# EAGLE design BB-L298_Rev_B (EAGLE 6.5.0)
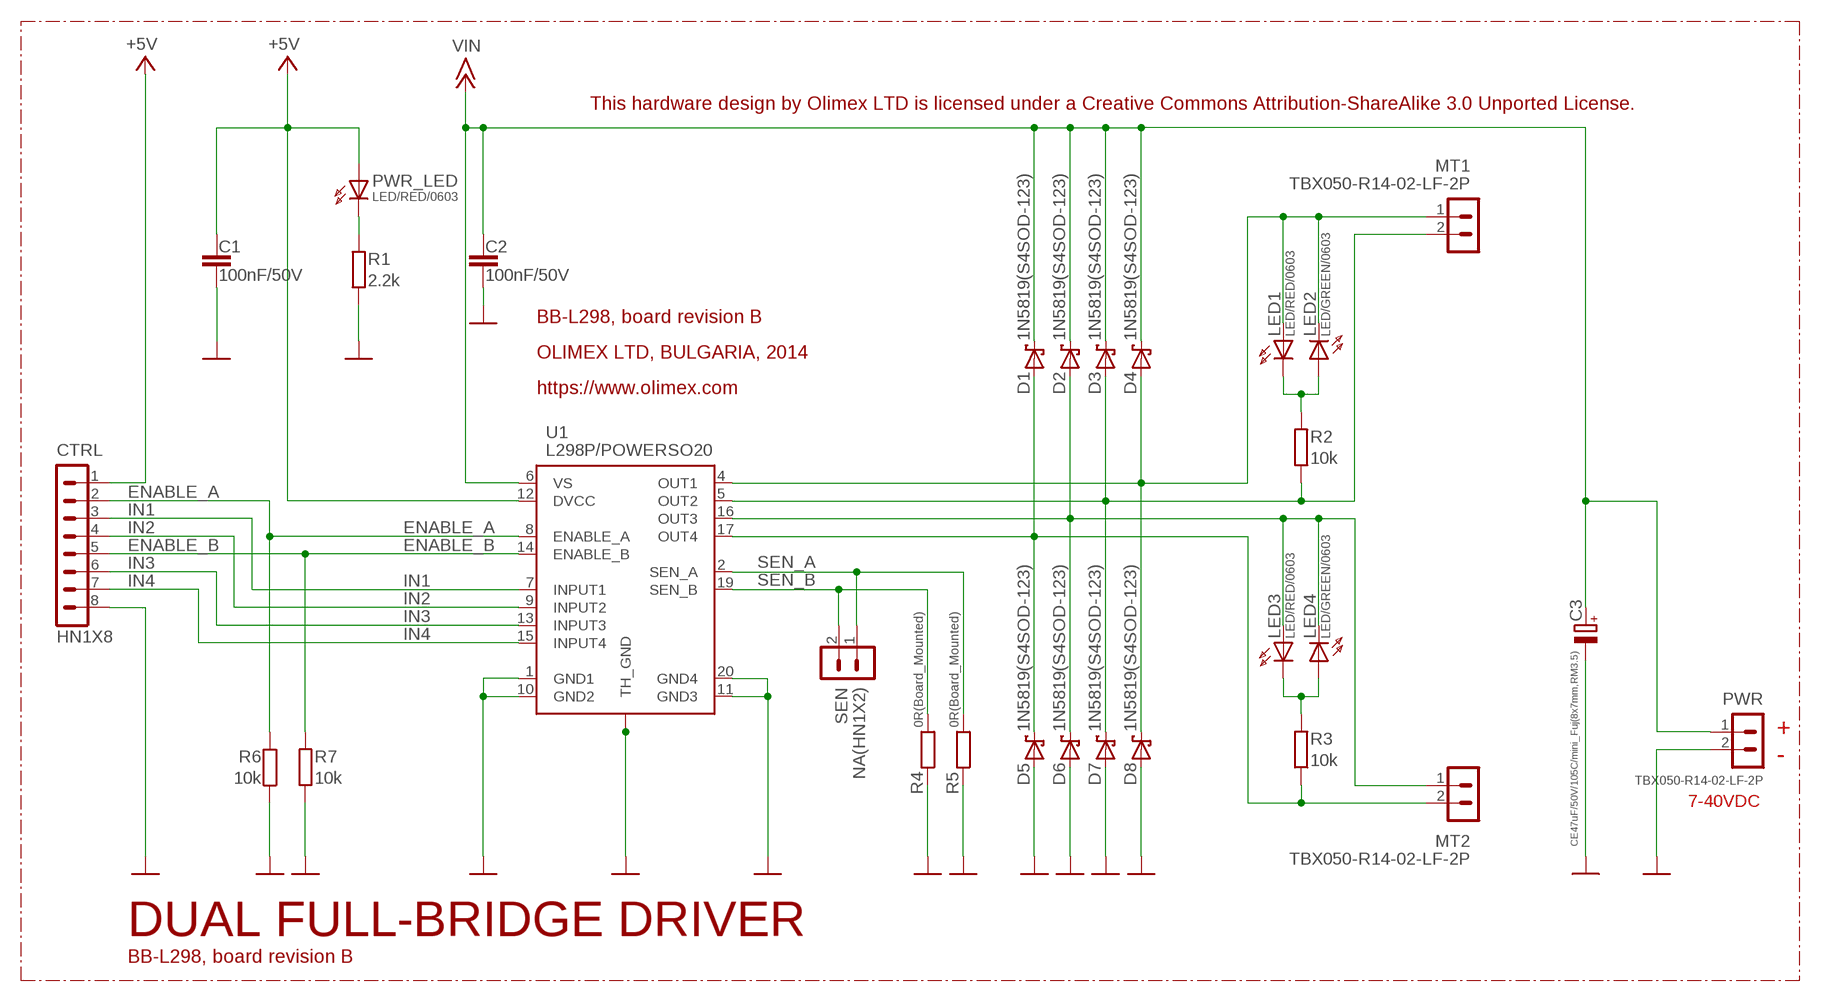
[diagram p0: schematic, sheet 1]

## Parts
C1  100nF/50V  C-EUC0603_DWS  [C0603_DWS]
C2  100nF/50V  C-EUC0603_DWS  [C0603_DWS]
C3  CE47uF/50V/105C/mini_Fuj(8x7mm,RM3.5)  CPOL-EUE3.5-8  [E3,5-8]
CTRL  HN1X8  CON8HN1X8  [HN1X8]
D1  1N5819(S4SOD-123)  SCHOTKKY7.62SS-1N5819(S4SOD-123)  [SOD-123]
D2  1N5819(S4SOD-123)  SCHOTKKY7.62SS-1N5819(S4SOD-123)  [SOD-123]
D3  1N5819(S4SOD-123)  SCHOTKKY7.62SS-1N5819(S4SOD-123)  [SOD-123]
D4  1N5819(S4SOD-123)  SCHOTKKY7.62SS-1N5819(S4SOD-123)  [SOD-123]
D5  1N5819(S4SOD-123)  SCHOTKKY7.62SS-1N5819(S4SOD-123)  [SOD-123]
D6  1N5819(S4SOD-123)  SCHOTKKY7.62SS-1N5819(S4SOD-123)  [SOD-123]
D7  1N5819(S4SOD-123)  SCHOTKKY7.62SS-1N5819(S4SOD-123)  [SOD-123]
D8  1N5819(S4SOD-123)  SCHOTKKY7.62SS-1N5819(S4SOD-123)  [SOD-123]
LED1  LED/RED/0603  LED0603DWS  [LED-0603]
LED2  LED/GREEN/0603  LED0603DWS  [LED-0603]
LED3  LED/RED/0603  LED0603DWS  [LED-0603]
LED4  LED/GREEN/0603  LED0603DWS  [LED-0603]
MT1  TBX050-R14-02-LF-2P  CON2_TBX050-R14-02-LF-2P  [TBX050-R14-02-LF-2P]
MT2  TBX050-R14-02-LF-2P  CON2_TBX050-R14-02-LF-2P  [TBX050-R14-02-LF-2P]
PWR  TBX050-R14-02-LF-2P  CON2_TBX050-R14-02-LF-2P  [TBX050-R14-02-LF-2P]
PWR_LED  LED/RED/0603  LED0603DWS  [LED-0603]
R1  2.2k  R-EU_R0603_5MIL_DWS  [R0603_5MIL_DWS]
R2  10k  R-EU_R0603_5MIL_DWS  [R0603_5MIL_DWS]
R3  10k  R-EU_R0603_5MIL_DWS  [R0603_5MIL_DWS]
R4  0R(Board_Mounted)  R-EU_R1206_5MIL_WS  [R1206_5MIL_WS]
R5  0R(Board_Mounted)  R-EU_R1206_5MIL_WS  [R1206_5MIL_WS]
R6  10k  R-EU_R0603_5MIL_DWS  [R0603_5MIL_DWS]
R7  10k  R-EU_R0603_5MIL_DWS  [R0603_5MIL_DWS]
SEN  NA(HN1X2)  CON2HN1X2  [HN1X2]
U1  L298P/POWERSO20  [POWRESO-20_THERM]

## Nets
+5V: C1.2 CTRL.1 PWR_LED.A U1.12(DVCC)
+15V: C2.2 C3.+ D1.C D2.C D3.C D4.C PWR.1 U1.6(VS) ; supply symbol labelled VIN
ENABLE_A: CTRL.2 R6.2 U1.8(ENABLE_A)
ENABLE_B: CTRL.5 R7.2 U1.14(ENABLE_B)
GND [pwr]: C1.1 C2.1 C3.- CTRL.8 D5.A D6.A D7.A D8.A PWR.2 R1.1 R4.1 R5.1 R6.1 R7.1 U1.1(GND1) U1.10(GND2) U1.11(GND3) U1.20(GND4) U1.THERM_GND1(TH_GND) U1.THERM_GND2 U1.THERM_GND3 U1.THERM_GND4 U1.THERM_GND5 U1.THERM_GND6 U1.THERM_GND7
IN1: CTRL.3 U1.7(INPUT1)
IN2: CTRL.4 U1.9(INPUT2)
IN3: CTRL.6 U1.13(INPUT3)
IN4: CTRL.7 U1.15(INPUT4)
N$1: LED1.C LED2.A R2.2
N$2: LED3.C LED4.A R3.2
N$3: PWR_LED.C R1.2
OUT1: D4.A D8.C LED1.A LED2.C MT1.1 U1.4(OUT1)
OUT2: D3.A D7.C MT1.2 R2.1 U1.5(OUT2)
OUT3: D2.A D6.C LED3.A LED4.C MT2.1 U1.16(OUT3)
OUT4: D1.A D5.C MT2.2 R3.1 U1.17(OUT4)
SEN_A: R5.2 SEN.1 U1.2(SEN_A)
SEN_B: R4.2 SEN.2 U1.19(SEN_B)

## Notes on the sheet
- This hardware design by Olimex LTD is licensed under a Creative Commons Attribution-ShareAlike 3.0 Unported License.
- BB-L298, board revision B
- OLIMEX LTD, BULGARIA, 2014
- https://www.olimex.com
- +
- -
- 7-40VDC
- DUAL FULL-BRIDGE DRIVER
- BB-L298, board revision B

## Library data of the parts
C1 C2 = rcl:C-EU: CAPACITOR, European symbol
C3 = rcl:CPOL-EU: POLARIZED CAPACITOR, European symbol
CTRL = Penko:CON8
D1-D8 = gogo:SCHOTKKY7.62SS
LED1-LED4 PWR_LED = DOUBLE-SIDE:LED
MT1 MT2 PWR SEN = Penko:CON2
R1-R7 = rcl:R-EU_: RESISTOR, European symbol
U1 = st-microelectronics:L298P

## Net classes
0 default: width 0.254 mm, drill 0.6 mm, clearance 0.254 mm
1 pwr: width 0.25 mm
2 thin: width 0.025 mm, clearance 0.025 mm
3 gsm_pwr: width 0.914 mm, drill 0.787 mm

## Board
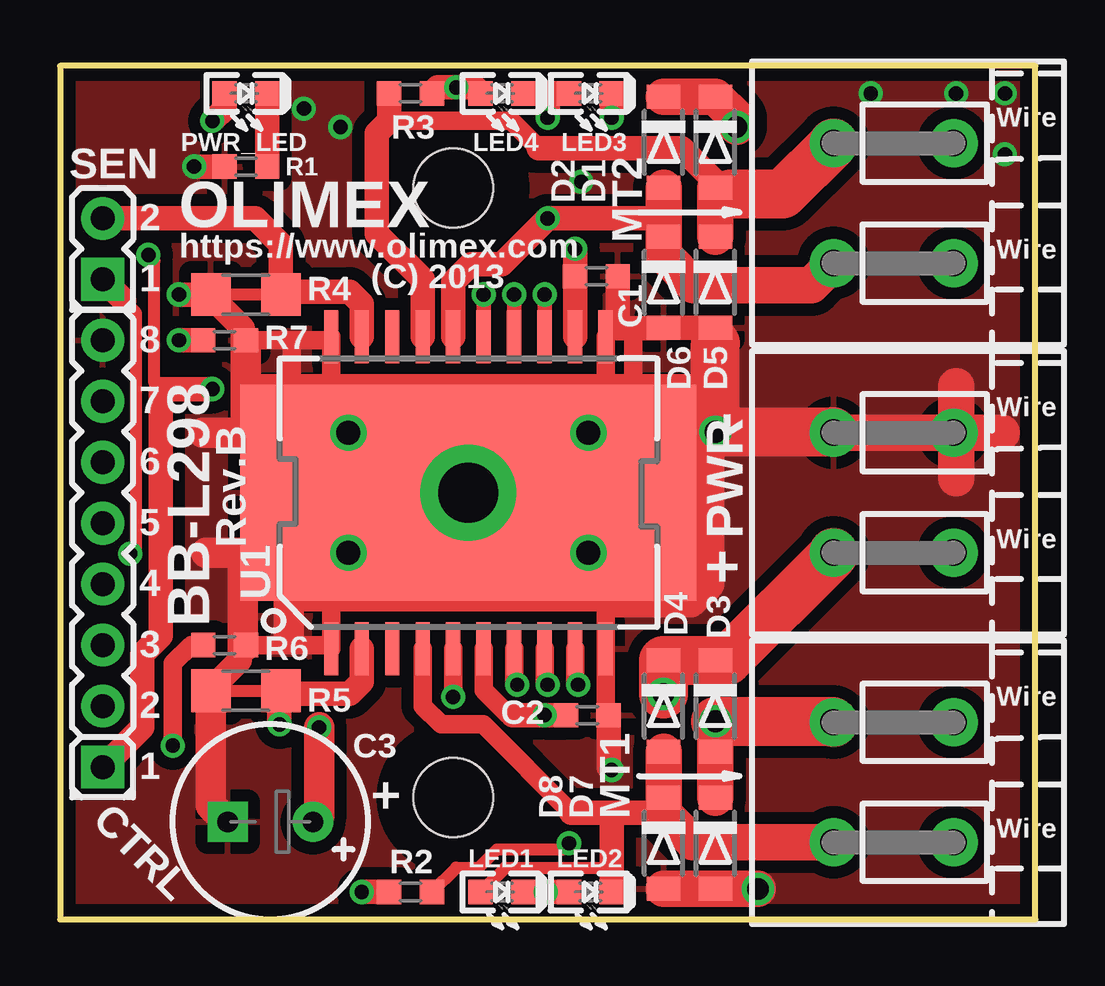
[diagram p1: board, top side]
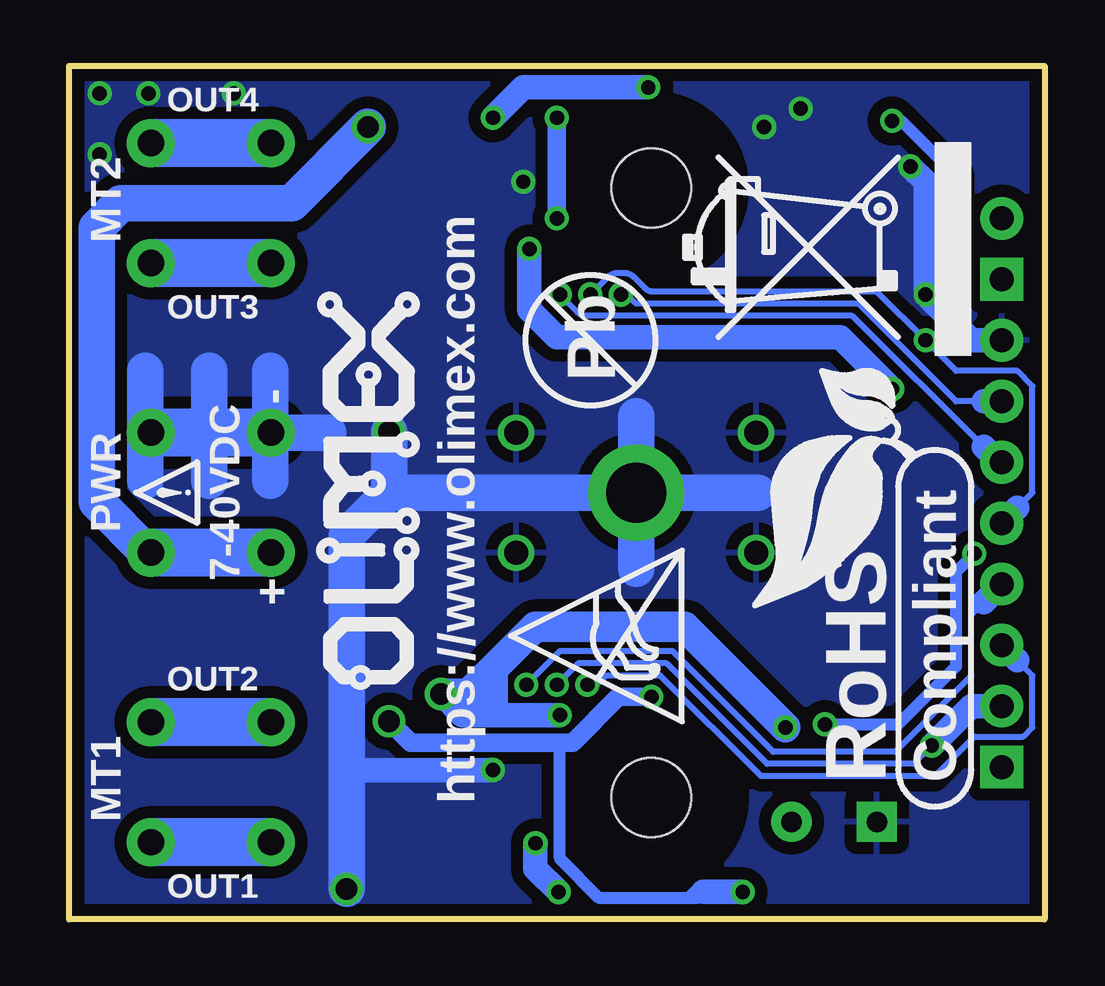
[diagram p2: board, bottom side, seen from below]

Size 40.64 x 35.56 mm. Coordinates in mm from the lower left corner, seen from the top.
Outline: 0,0 40.64,0 40.64,35.56 0,35.56 0,0
Copper layers (1+16): Top 0.035mm / dielectric 1.5mm / Bottom 0.035mm
Design rules "default": minimum track width 9.5mil, minimum drill 23mil, track to track 9.5mil, track to pad 9.5mil, pad to pad 9.5mil, via to via 10mil, smd to smd 1mil, copper to edge 10mil, drill to drill 8mil, minimum pad ring 10mil, minimum via ring 8mil, stop-mask expansion 4mil, vias tented up to drill 40mil, thermal gap 20mil
Holes 3.3 mm at 16.38,30.48 16.38,5.08
tRestrict: area 13.8,27.9 to 18.9,33; area 13.8,2.5 to 18.9,7.6; 2 lines
bRestrict: area 13,27.1 to 19.8,33.9; area 13,1.7 to 19.8,8.5

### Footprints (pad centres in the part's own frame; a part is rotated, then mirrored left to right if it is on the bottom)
C0603_DWS = smd 1.016 x 1.016: 1 -0.889,0; 2 0.889,0
E3,5-8 = drill 0.864 pad 1.676: + -1.778,0 | drill 0.864 pad 1.676 square: - 1.778,0
HN1X8 = drill 1 pad 1.778 square: 1 -8.89,0 | drill 1 pad 1.778: 2 -6.35,0; 3 -3.81,0; 4 -1.27,0; 5 1.27,0; 6 3.81,0; 7 6.35,0; 8 8.89,0
SOD-123 = smd 1 x 1.4: A 1.9,0; C -1.9,0
LED-0603 = smd 1.016 x 1.016: A 0.889,0; C -0.889,0
TBX050-R14-02-LF-2P = drill 1.1 pad 2: 1 -2.5,3.2; 2 2.5,3.2; 3 -2.5,-1.8; 4 2.5,-1.8
R0603_5MIL_DWS = smd 1.016 x 1.016: 1 -0.889,0; 2 0.889,0
R1206_5MIL_WS = smd 1.651 x 1.778: 1 -1.46,0; 2 1.46,0
HN1X2 = drill 1 pad 1.778 square: 1 -1.27,0 | drill 1 pad 1.778: 2 1.27,0
POWRESO-20_THERM = smd 0.6 x 2.2: 1 -5.715,-6.5; 2 -4.445,-6.5; 3 -3.175,-6.5; 4 -1.905,-6.5; 5 -0.635,-6.5; 6 0.635,-6.5; 7 1.905,-6.5; 8 3.175,-6.5; 9 4.445,-6.5; 10 5.715,-6.5; 11 5.715,6.5; 12 4.445,6.5; 13 3.175,6.5; 14 1.905,6.5; 15 0.635,6.5; 16 -0.635,6.5; 17 -1.905,6.5; 18 -3.175,6.5; 19 -4.445,6.5; 20 -5.715,6.5 | smd 10 x 9: THERM_GND1 -4.5,0; THERM_GND2 4.5,0 | drill 2.5 pad 4: THERM_GND3 0,0 | drill 1: THERM_GND4 -5,2.5; THERM_GND5 -5,-2.5; THERM_GND6 5,2.5; THERM_GND7 5,-2.5

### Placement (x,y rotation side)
C1  22.35,26.8 180 top
C2  21.97,8.51 180 top
C3  8.76,4.06 180 top
CTRL  1.78,15.24 90 top
D1  27.3,32.38 270 top
D2  25.15,32.38 270 top
D3  27.3,8.89 270 top
D4  25.15,8.89 270 top
D5  27.3,26.54 270 top
D6  25.15,26.54 270 top
D7  27.3,3.17 270 top
D8  25.15,3.17 270 top
LED1  18.42,1.14 180 top
LED2  22.1,1.14 180 top
LED3  22.1,34.42 180 top
LED4  18.42,34.42 180 top
MT1  35.43,5.71 90 top
MT2  35.43,29.84 90 top
PWR  35.43,17.78 90 top
PWR_LED  7.75,34.42 180 top
R1  7.75,31.37 0 top
R2  14.6,1.14 0 top
R3  14.6,34.42 0 top
R4  7.75,26.04 0 top
R5  7.75,9.53 0 top
R6  6.86,11.43 180 top
R7  6.86,24.13 180 top
SEN  1.78,27.94 90 top
U1  17.02,17.78 0 top
U$1  [ATTENTION_SMALL]  35.31,16.51 90 bottom
U$3  [RECYCLE_BIN1/4]  3.05,23.5 90 bottom
U$5  [ESD_SYMBOL]  15.11,8.26 90 bottom
U$6  [PB]  18.92,24.13 90 bottom
U$13  [ROHS]  3.68,5.71 90 bottom
U$14  [OLIMEX1_V]  25.91,27.3 90 bottom

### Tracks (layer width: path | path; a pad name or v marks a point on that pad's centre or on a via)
+5V  (via drill 0.6)
  Top 0.508: 4.19,22.1 3.94,22.35 3.94,27.43 v3.68,27.69
  Top 1.016: U1.12 C1.2 v21.46,27.94 | CTRL.1 3.43,8 3.43,11.05 4.19,11.81 4.19,22.1 v6.35,22.1 | v6.35,33.27 6.86,33.78 PWR_LED.A
  Bottom 0.508: v6.35,33.27 5.97,33.27 3.68,30.99 v3.68,27.69
  Bottom 1.016: v21.46,27.94 21.46,25.4 20.32,24.26 8.51,24.26 v6.35,22.1
+15V  (via drill 0.6, 0.9)
  Top 0.762: U1.6 17.65,9.55 18.69,8.51 18.87,8.51
  Top 1.016: 18.87,8.51 v20.19,8.51 C2.2
  Top 1.27: C3.+ 10.79,4.32 v10.79,8
  Top 1.524: v28.19,33.02 28.19,33.4 D1.C D2.C
  Top 2.032: v25.15,9.4 D4.C D3.C 27.81,10.79 32.23,15.21 PWR.1
  Bottom 0.762: 22.73,10.67 22.73,8.51 23.75,9.53 23.88,9.53
  Bottom 1.016: 23.11,8.51 24,9.4 | 23.11,8.51 22.73,8.51 v20.19,8.51 | 23.11,8.51 24.26,8.51 v25.15,9.4
  Bottom 1.27: v25.15,9.4 24,9.4 23.88,9.53 22.73,10.67 21.21,12.19 14.99,12.19 v10.79,8
  Bottom 1.524: PWR.1 37.38,15.28 39.5,17.4 39.5,28.83 38.48,29.84 31.37,29.84 v28.19,33.02
ENABLE_A  (via drill 0.6)
  Top 0.762: v20.32,9.78 20.19,9.91 U1.8 | R6.2 5.46,11.43 4.7,10.67 v4.7,7.24
  Bottom 0.254: v20.32,9.78 19.43,10.67 15.75,10.67 11.56,6.48 5.46,6.48 v4.7,7.24
  Bottom 1.016: CTRL.2 3.05,8.89 v4.7,7.24
ENABLE_B  (via drill 0.6)
  Top 0.61: v18.92,26.04 U1.14
  Top 1.016: v4.95,24.13 R7.2
  Bottom 0.254: v18.92,26.04 18.18,26.77 arc45 17.82,26.92 17.48,26.92 arc45 17.12,26.77 16.66,26.31 arc-45 16.3,26.16 6.99,26.16 v4.95,24.13 3.68,22.86 1.14,22.86 0.51,22.23 0.51,17.78 1.14,17.14
  Bottom 1.016: CTRL.5 1.14,17.14
GND  (via drill 0.6, 0.9)
  Top 0.508: U1.11 22.73,24.64 23.24,24.64
  Top 0.762: C2.1 22.73,8.64 U1.10 22.73,13.46 | R6.1 9.52,11.43 | 9.52,11.43 9.52,11.68 | 9.52,11.43 11.3,11.43 | 11.3,11.43 U1.1 | 11.3,24.13 9.65,24.13 | 9.65,24.13 R7.1 | 11.3,11.43 11.3,13.46 | 22.73,22.23 U1.11 | 11.3,22.23 11.3,24.13 | 11.3,24.13 U1.20 | 9.65,22.23 9.65,24.13 | 23.88,24.64 23.88,22.23
  Top 1.016: 27.3,24 D5.A D6.A 23.88,24.64 23.24,24.64 C1.1 | v22.99,6.22 22.86,6.35 C2.1 | R5.1 6.29,9.59 7.49,10.79 7.49,11.43 7.62,11.43 | R7.1 7.62,24.26 7.62,24.64 6.29,25.97 R4.1 v4.95,26.04 | v5.59,31.37 R1.1 | 26.92,22.23 23.88,22.23 22.73,22.23 11.3,22.23 9.65,22.23 7.75,22.23
  Top 1.27: 7.62,15.28 U1.THERM_GND5 | R6.1 7.62,11.43 7.62,15.28 | 7.62,15.28 6.1,15.28 | R5.1 6.29,4.76 C3.- | 7.75,20.28 U1.THERM_GND4 | R7.1 7.75,22.23 7.75,20.28 | 7.75,20.28 5.97,20.28 | 27.05,20.32 27.05,13.97 26.29,13.21 22.99,13.21 22.73,13.46 11.3,13.46 9.52,13.46 9.52,11.68
  Top 1.524: D8.A D7.A 28.07,1.27 28.08,1.27 v29.08,1.27 | PWR.2 37.34,20.28 | 37.34,20.28 37.34,18.38 | 37.34,20.28 39.24,20.28 | 37.34,20.28 37.34,22.23
  Top 2.032: U1.THERM_GND6 22.06,20.32 27.05,20.32 v27.3,20.32 | PWR.2 32.19,20.32 v27.3,20.32 | v27.3,20.32 27.3,24
  Bottom 1.016: v22.99,6.22 29.08,6.22 | CTRL.8 3.05,24.13 v4.95,26.04 4.95,30.73 v5.59,31.37
  Bottom 1.524: v27.3,20.32 27.3,17.78 | U1.THERM_GND3 11.94,17.78 | U1.THERM_GND3 17.02,20.95 | U1.THERM_GND3 17.02,14.61 | 27.3,17.78 U1.THERM_GND3 | 27.3,17.78 29.08,16 29.08,6.22 v29.08,1.27 | 29.85,20.28 PWR.2 32.26,20.28 | 32.26,20.28 32.26,22.86 | 32.26,20.28 32.26,18.29 | 32.26,20.28 34.8,20.28 | 34.8,20.28 37.46,20.28 | 37.46,20.28 37.46,18.29 | 37.46,20.28 37.46,22.86 | 34.8,20.28 34.8,22.86 | 34.8,20.28 34.8,18.29
  other vias: 10.16,33.78 21.72,30.73 11.68,33.02 33.78,34.42 39.37,34.42 37.34,34.42 39.37,31.88
  pour Bottom (isolate 0.508, rank 4): 45.59,38.1 -2.67,38.1 -2.67,-2.54 45.59,-2.54
  pour Top (isolate 0.508, rank 4): -5.21,40.64 48.13,40.64 48.13,-5.08 -5.21,-5.08
IN1  (via drill 0.6)
  Top 0.762: v19.05,9.78 18.92,9.91 U1.7
  Bottom 0.254: v19.05,9.78 18.67,9.78 18.29,10.16 16,10.16 11.81,5.97 4.57,5.97 2.92,7.62 0.89,7.62 0.51,8 0.51,10.16 1.14,10.79
  Bottom 1.016: 1.14,10.79 CTRL.3
IN2  (via drill 0.6)
  Top 0.762: v21.59,9.78 21.46,9.91 U1.9
  Bottom 0.254: v21.59,9.78 20.19,11.18 15.49,11.18 11.3,6.99 6.22,6.99 3.05,10.16 3.05,12.7 2.54,13.21
  Bottom 1.016: 2.54,13.21 CTRL.4
IN3  (via drill 0.6)
  Top 0.61: v20.19,26.04 U1.13
  Bottom 0.254: 2.54,19.68 8,25.15 19.09,25.15 arc45 19.45,25.3 v20.19,26.04
  Bottom 1.016: CTRL.6 1.91,19.05 2.54,19.68
IN4  (via drill 0.6)
  Top 0.61: v17.65,26.04 U1.15
  Bottom 0.254: 2.54,21.59 3.68,21.59 7.75,25.65 17.02,25.65 17.4,26.04 v17.65,26.04
  Bottom 1.016: CTRL.7 2.54,21.59
N$1  (via drill 0.6)
  Top 0.508: R2.2 16.51,2.16 17.45,2.16 18.21,2.92 20.96,2.92 v21.21,3.17
  Top 1.016: LED2.A v20.24,1.14 LED1.C
  Bottom 1.016: v20.24,1.14 21.21,2.11 v21.21,3.17
N$2  (via drill 0.6)
  Top 1.016: v22.99,33.4 LED3.C | LED4.A 17.27,34.67 v16.51,34.67 15.75,34.67 R3.2
  Bottom 1.016: v22.99,33.4 21.72,34.67 v16.51,34.67
N$3
  Top 1.016: R1.2 PWR_LED.C
OUT1
  Top 0.508: LED1.A 18.54,2.16 22.99,2.16
  Top 0.762: U1.4 15.11,8.89 15.87,8.13 17.63,8.13 21.31,4.45
  Top 1.016: LED2.C 22.99,2.16 22.99,4.45 | 22.99,4.45 21.31,4.45 | 22.99,4.45 25.15,4.45
  Top 1.524: MT1.1 26.38,3.21 25.15,4.45 D8.C D4.A
OUT2  (via drill 0.6, 0.9)
  Top 0.762: v16.38,9.27 U1.5
  Top 1.016: R2.1 v12.57,1.14
  Top 1.524: D7.C D3.A v27.3,8.26
  Top 2.032: MT1.2 32.19,8.26 v27.3,8.26
  Bottom 0.508: 14.22,1.14 14.48,0.89 14.83,0.89 | 14.83,0.89 18.54,0.89 20.19,2.54 20.19,7.37 | 14.83,0.89 14.58,1.14
  Bottom 0.762: v16.38,9.27 17.76,9.27 19.66,7.37 20.19,7.37 26.42,7.37 v27.3,8.26
  Bottom 1.016: v12.57,1.14 14.22,1.14
OUT3  (via drill 0.6)
  Top 1.016: U1.16 16.38,26.57 17.12,27.3 18.42,27.3 v20.32,29.21 25.15,29.21 | 20.32,34.42 LED4.C | 20.32,34.42 LED3.A | v20.32,33.4 20.32,34.42
  Top 1.524: MT2.1 31.3,26.42 26.42,26.42 25.15,27.69 D6.C 25.15,29.21 D2.A
  Bottom 0.762: v20.32,29.21 v20.32,33.4
OUT4
  Top 0.762: 19.94,32.13 18.8,33.27 13.72,33.27
  Top 1.016: U1.17 15.11,26.67 13.21,28.57 13.21,32.77 13.72,33.27 R3.1 | D1.A 27.3,30.73 25.91,32.13 19.94,32.13
  Top 1.524: D1.A 27.3,30.23 | 27.3,30.23 D5.C | 27.3,30.23 27.94,30.23
  Top 2.032: MT2.2 30.11,30.23 27.94,30.23
SEN_A  (via drill 0.6)
  Top 0.508: 2.67,25.78 3.17,25.27 3.17,15.49 v2.92,15.24 | 6.86,9.53 R5.2
  Top 1.016: U1.2 12.57,9.91 12.06,9.4 9.21,9.4 R5.2 9.14,9.46 v9.14,8.13 | 2.67,25.78 SEN.1
  Bottom 0.508: v2.92,15.24 3.68,14.48 3.68,10.54 6.1,8.13 v9.14,8.13
SEN_B
  Top 0.508: R4.2 6.99,26.04
  Top 1.016: 9.21,26.16 12.06,26.16 12.57,25.65 U1.19 | 9.21,26.16 R4.2 | SEN.2 8.13,29.21 9.21,28.13 9.21,26.16

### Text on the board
Top: Total Errors: 64
tNames: 2 | OLIMEX | https://www.olimex.com | 1 | (C) 2013 | 8 | 7 | - | 6 | 5 | Rev.B | + | 4 | BB-L298 | 3 | 2 | 1 | +
bNames: OUT4 | OUT3 | - | 7-40VDC | + | OUT2 | https://www.olimex.com | OUT1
